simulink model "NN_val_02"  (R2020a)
settings: Solver=ode45  StartTime=0.0  StopTime=1000  RelTol=1e-3  EnableMultiTasking=on
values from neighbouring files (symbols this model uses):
  Ts = 0.05    [init_model.m]
libraries: neural x26

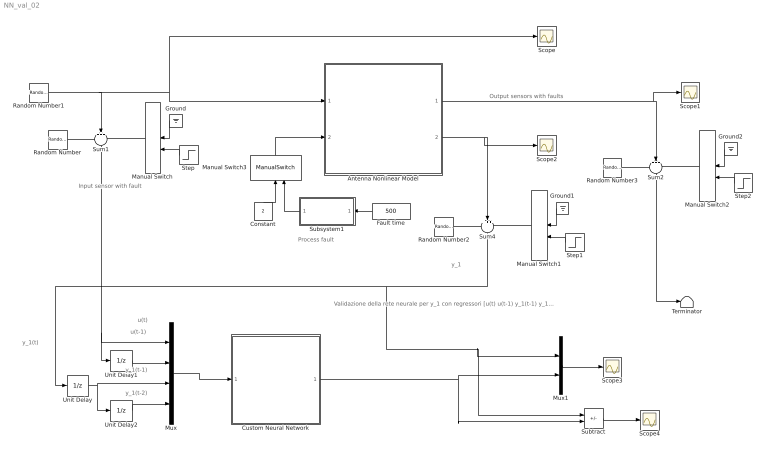
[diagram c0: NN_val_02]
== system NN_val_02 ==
  note: Validazione della rete neurale per y_1 con regressori [u(t) u(t-1) y_1(t-1) y_1(t-2)]
  note: y_1(t)
  note: y_1(t-1)
  note: y_1
  note: u(t)
  note: Output sensors with faults
  note: Process fault
  note: Input sensor with fault
  note: u(t-1)
  note: y_1(t-2)
  Antenna Nonlinear Model : Subsystem
  Constant : Constant  Value=2
  Custom Neural Network : Subsystem
      mask help: Custom Neural Network
  Fault time : Constant  Value=500
  Ground : Ground
  Ground1 : Ground
  Ground2 : Ground
  Manual Switch{,1..3} (4 alike) : ManualSwitch
  Mux : Mux
  Mux1 : Mux  Inputs=2
  Random Number : RandomNumber  Variance=0.0001  Seed=1  SampleTime=Ts
  Random Number1 : RandomNumber  Variance=0.1  SampleTime=10
  Random Number2 : RandomNumber  Variance=0.00001  Seed=2  SampleTime=Ts
  Random Number3 : RandomNumber  Variance=0.00001  Seed=3  SampleTime=Ts
  Scope{,1..4} (5 alike) : Scope
  Step : Step  Time=500  SampleTime=0
  Step1 : Step  Time=500  SampleTime=0
  Step2 : Step  Time=50  SampleTime=0
  Subsystem1 : Subsystem
  Subtract : Sum  Inputs=+-
  Sum1 : Sum  Inputs=+++  SaturateOnIntegerOverflow=on
  Sum2 : Sum  Inputs=+++  SaturateOnIntegerOverflow=on
  Sum4 : Sum  Inputs=+++  SaturateOnIntegerOverflow=on
  Terminator : Terminator
  Unit Delay : UnitDelay  SampleTime=Ts  HasFrameUpgradeWarning=on
  Unit Delay1 : UnitDelay  SampleTime=Ts  HasFrameUpgradeWarning=on
  Unit Delay2 : UnitDelay  SampleTime=Ts  HasFrameUpgradeWarning=on
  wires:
  Random Number1/1 -> Scope/1, Antenna Nonlinear Model/1(force), Sum1/2
  Random Number/1 -> Sum1/1
  Manual Switch/1 -> Sum1/3
  Sum1/1 -> Unit Delay1/1, Mux/1
  Ground/1 -> Manual Switch/1
  Step/1 -> Manual Switch/2
  Random Number2/1 -> Sum4/1
  Ground1/1 -> Manual Switch1/1
  Manual Switch1/1 -> Sum4/3
  Step1/1 -> Manual Switch1/2
  Antenna Nonlinear Model/2(velocity) -> Sum4/2, Scope2/1
  Random Number3/1 -> Sum2/1
  Ground2/1 -> Manual Switch2/1
  Manual Switch2/1 -> Sum2/3
  Step2/1 -> Manual Switch2/2
  Antenna Nonlinear Model/1(angle) -> Sum2/2, Scope1/1
  Sum2/1 -> Terminator/1
  Fault time/1 -> Subsystem1/1(Fault time)
  Subsystem1/1(Fault) -> Manual Switch3/2
  Manual Switch3/1 -> Antenna Nonlinear Model/2(drag)
  Constant/1 -> Manual Switch3/1
  Mux/1 -> Custom Neural Network/1(Input)
  Unit Delay1/1 -> Mux/2
  Unit Delay/1 -> Unit Delay2/1, Mux/3
  Unit Delay2/1 -> Mux/4
  Mux1/1 -> Scope3/1
  Custom Neural Network/1(Output) -> Subtract/2, Mux1/2
  Sum4/1 -> Mux1/1, Subtract/1, Unit Delay/1
  Subtract/1 -> Scope4/1

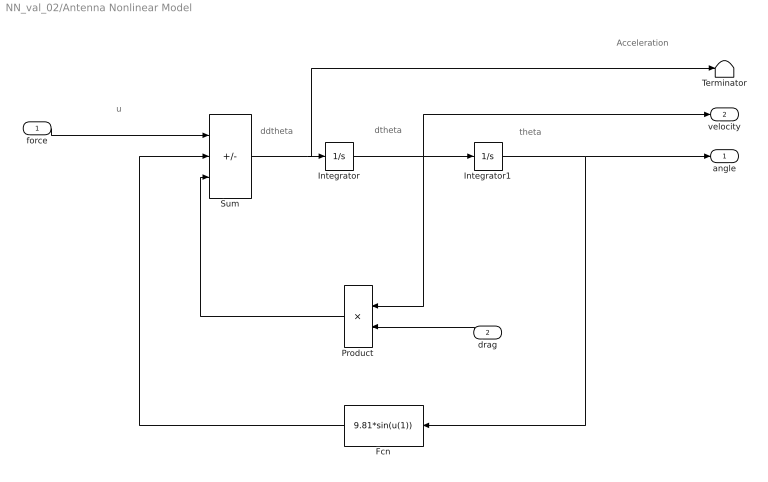
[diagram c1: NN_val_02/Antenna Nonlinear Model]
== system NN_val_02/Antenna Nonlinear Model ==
  note: Acceleration
  note: ddtheta
  note: dtheta
  note: theta
  note: u
  force : Inport
  drag : Inport  Port=2
  Fcn : Fcn  Expr=9.81*sin(u(1))
  Integrator : Integrator
  Integrator1 : Integrator  InitialCondition=(pi/180)*90
  Product : Product
  Sum : Sum  Inputs=+--  SaturateOnIntegerOverflow=on
  Terminator : Terminator
  angle : Outport
  velocity : Outport  Port=2
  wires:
  Sum/1 -> Terminator/1, Integrator/1
  Integrator/1 -> Product/1, Integrator1/1, velocity/1
  Integrator1/1 -> angle/1, Fcn/1
  Fcn/1 -> Sum/2
  Product/1 -> Sum/3
  force/1 -> Sum/1
  drag/1 -> Product/2

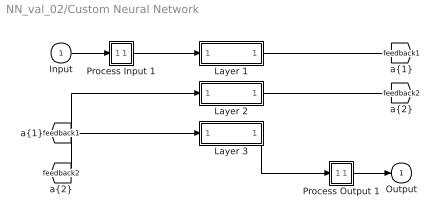
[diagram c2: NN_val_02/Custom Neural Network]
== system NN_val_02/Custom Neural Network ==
  Input : Inport  PortDimensions=4  SampleTime=0.05
  Layer 1 : Subsystem
  Layer 2 : Subsystem
  Layer 3 : Subsystem
  Process Input 1 : Subsystem
  Process Output 1 : Subsystem
  Output : Outport  InitialOutput=0
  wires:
  Input/1 -> Process Input 1/1(x)
  Process Output 1/1(y) -> Output/1
  Process Input 1/1(p) -> Layer 1/1("p{1}")
  Layer 1/1("a{1}") -> [feedback1]
  [feedback1] -> Layer 2/1("a{1} ")
  Layer 2/1("a{2}") -> [feedback2]
  [feedback2] -> Layer 3/1("a{2} ")
  Layer 3/1("a{3}") -> Process Output 1/1(a)

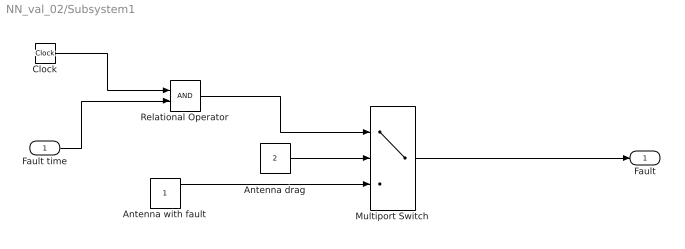
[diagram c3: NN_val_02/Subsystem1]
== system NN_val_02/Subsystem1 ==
  Fault time : Inport
  Antenna drag : Constant  Value=2
  Antenna with fault : Constant
  Clock : Clock
  Multiport Switch : MultiPortSwitch  DataPortOrder=Zero-based contiguous  Inputs=2  zeroidx=on
  Relational Operator : RelationalOperator  OutDataTypeStr=boolean  RndMeth=Simplest
  Fault : Outport
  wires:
  Clock/1 -> Relational Operator/1
  Fault time/1 -> Relational Operator/2
  Antenna drag/1 -> Multiport Switch/2
  Relational Operator/1 -> Multiport Switch/1
  Multiport Switch/1 -> Fault/1
  Antenna with fault/1 -> Multiport Switch/3

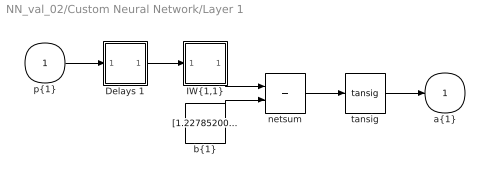
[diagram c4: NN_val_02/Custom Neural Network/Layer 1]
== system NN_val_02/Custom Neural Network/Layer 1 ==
  "p{1}" : Inport  PortDimensions=4  SampleTime=0.05
  Delays 1 : Subsystem
  "IW{1,1}" : Subsystem
  "b{1}" : Constant  Value=[1.227852000795871756366750560118816792964935302734375;-1.2068086972006153434477937480551190674304962158203125;-0.469116205279137721273485794881707988679409027099609375;0.537033543120907008727726861252449452877044677734375;0.68757712323574382562441087429760955274105072021484375;-2.165370420921475247411080999881960451602935791015625;-3.80990414820139111640173723571933805942535400390625]
  netsum : Sum  Inputs=2  InputSameDT=on  SaturateOnIntegerOverflow=on
  tansig : neural/Transfer Functions/tansig
  "a{1}" : Outport  InitialOutput=[0;0;0;0;0;0;0]
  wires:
  "p{1}"/1 -> Delays 1/1("p{1}")
  Delays 1/1("pd{1,1}") -> "IW{1,1}"/1("pd{1,1}")
  "IW{1,1}"/1("iz{1,1}") -> netsum/1
  "b{1}"/1 -> netsum/2
  netsum/1 -> tansig/1
  tansig/1 -> "a{1}"/1

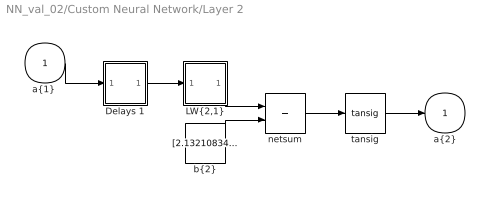
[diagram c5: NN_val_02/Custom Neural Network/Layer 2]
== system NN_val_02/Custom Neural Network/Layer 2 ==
  "a{1} " : Inport  PortDimensions=7  SampleTime=0.05
  Delays 1 : Subsystem
  "LW{2,1}" : Subsystem
  "b{2}" : Constant  Value=[2.132108348660313179578906783717684447765350341796875;2.220142305818061601030422025360167026519775390625;-1.5267770156364133260495918875676579773426055908203125;1.3641049967075142834715961726033128798007965087890625;0.80441149195895922385801668497151695191860198974609375;0.245980875629058015618966237525455653667449951171875;-0.5502430248009293478617109940387308597564697265625;0.187105156518366344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
  netsum : Sum  Inputs=2  InputSameDT=on  SaturateOnIntegerOverflow=on
  tansig : neural/Transfer Functions/tansig
  "a{2}" : Outport  InitialOutput=[0;0;0;0;0;0;0;0;0;0;0;0;0;0;0]
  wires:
  "a{1} "/1 -> Delays 1/1("p{2}")
  Delays 1/1("pd{2,1}") -> "LW{2,1}"/1("ad{2,1}")
  "LW{2,1}"/1("lz{2,1}") -> netsum/1
  "b{2}"/1 -> netsum/2
  netsum/1 -> tansig/1
  tansig/1 -> "a{2}"/1

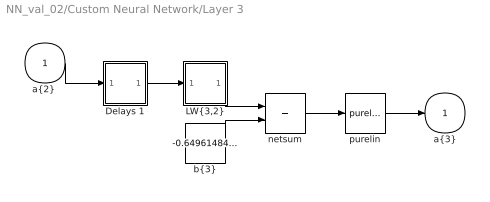
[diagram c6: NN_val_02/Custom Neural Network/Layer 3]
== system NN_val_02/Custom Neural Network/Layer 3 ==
  "a{2} " : Inport  PortDimensions=15  SampleTime=0.05
  Delays 1 : Subsystem
  "LW{3,2}" : Subsystem
  "b{3}" : Constant  Value=-0.64961484212074604993603088587406091392040252685546875
  netsum : Sum  Inputs=2  InputSameDT=on  SaturateOnIntegerOverflow=on
  purelin : neural/Transfer Functions/purelin
  "a{3}" : Outport  InitialOutput=0
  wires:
  "a{2} "/1 -> Delays 1/1("p{3}")
  Delays 1/1("pd{3,2}") -> "LW{3,2}"/1("ad{3,2}")
  "LW{3,2}"/1("lz{3,2}") -> netsum/1
  "b{3}"/1 -> netsum/2
  netsum/1 -> purelin/1
  purelin/1 -> "a{3}"/1

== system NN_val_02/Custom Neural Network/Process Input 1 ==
  x : Inport  PortDimensions=4  SampleTime=0.05
  p : Outport  PortDimensions=4  SampleTime=0.05
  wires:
  x/1 -> p/1

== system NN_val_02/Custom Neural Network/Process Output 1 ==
  a : Inport  PortDimensions=1  SampleTime=0.05
  y : Outport  PortDimensions=1  SampleTime=0.05
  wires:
  a/1 -> y/1

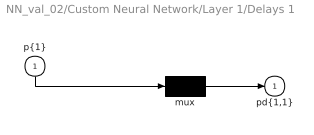
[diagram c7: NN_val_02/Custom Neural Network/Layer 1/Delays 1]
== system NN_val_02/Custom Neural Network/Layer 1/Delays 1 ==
  "p{1}" : Inport  PortDimensions=4  SampleTime=0.05
  mux : Mux  Inputs=1
  "pd{1,1}" : Outport
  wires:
  "p{1}"/1 -> mux/1
  mux/1 -> "pd{1,1}"/1

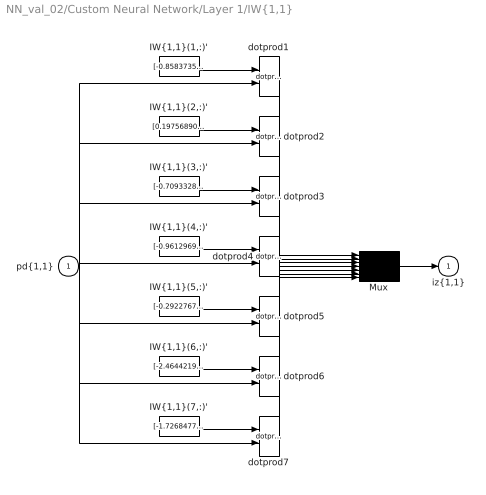
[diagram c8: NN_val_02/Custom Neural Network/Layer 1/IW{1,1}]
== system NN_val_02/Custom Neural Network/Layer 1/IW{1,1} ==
  "pd{1,1}" : Inport  PortDimensions=4  SampleTime=0.05
  "IW{1,1}(1,:)'" : Constant  Value=[-0.85837353691424123081077368624391965568065643310546875;-1.50167157946812235280731329112313687801361083984375;-1.2582699014576614882088279046001844108104705810546875;-0.81845080414747661823327007368789054453372955322265625]
  "IW{1,1}(2,:)'" : Constant  Value=[0.1975689051025306952613647126781870611011981964111328125;-1.1980691178201678948056496665230952203273773193359375;1.2091156479242730625855983817018568515777587890625;0.02637417164378029477145304326768382452428340911865234375]
  "IW{1,1}(3,:)'" : Constant  Value=[-0.7093328605358213412301893185940571129322052001953125;-2.107014242855214103400385283748619258403778076171875;-0.299913237321096204368586768396198749542236328125;-0.568643153566053438652261320385150611400604248046875]
  "IW{1,1}(4,:)'" : Constant  Value=[-0.96129696900881500543079027920612134039402008056640625;0.601804743455427892939724188181571662425994873046875;-0.7674148410687451349332377503742463886737823486328125;0.85896029266268880686396869350573979318141937255859375]
  "IW{1,1}(5,:)'" : Constant  Value=[-0.2922767950669269421126728047966025769710540771484375;0.2225160957405193096203532832078053615987300872802734375;0.8686197000875226503779913400649093091487884521484375;-0.279177521795706928831037885174737311899662017822265625]
  "IW{1,1}(6,:)'" : Constant  Value=[-2.464421946556701659147847749409265816211700439453125;-0.08884885706228863588851396571044460870325565338134765625;-0.27909020302141218650149312452413141727447509765625;0.422037319836571722664331218766164965927600860595703125]
  "IW{1,1}(7,:)'" : Constant  Value=[-1.7268477556460919419833999199909158051013946533203125;-0.1723568342494542215970199094954296015202999114990234375;-0.1833208379863790205011042644400731660425662994384765625;-0.6184209020560771374874775574426166713237762451171875]
  Mux : Mux  Inputs=7
  dotprod{1..7} (7 alike) : neural/Weight Functions/dotprod
  "iz{1,1}" : Outport
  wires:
  "IW{1,1}(1,:)'"/1 -> dotprod1/1
  "pd{1,1}"/1 -> dotprod1/2, dotprod2/2, dotprod3/2, dotprod4/2, dotprod5/2, dotprod6/2, dotprod7/2
  dotprod1/1 -> Mux/1
  "IW{1,1}(2,:)'"/1 -> dotprod2/1
  dotprod2/1 -> Mux/2
  "IW{1,1}(3,:)'"/1 -> dotprod3/1
  dotprod3/1 -> Mux/3
  "IW{1,1}(4,:)'"/1 -> dotprod4/1
  dotprod4/1 -> Mux/4
  "IW{1,1}(5,:)'"/1 -> dotprod5/1
  dotprod5/1 -> Mux/5
  "IW{1,1}(6,:)'"/1 -> dotprod6/1
  dotprod6/1 -> Mux/6
  "IW{1,1}(7,:)'"/1 -> dotprod7/1
  dotprod7/1 -> Mux/7
  Mux/1 -> "iz{1,1}"/1

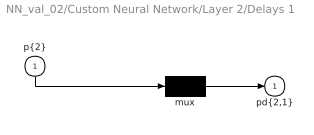
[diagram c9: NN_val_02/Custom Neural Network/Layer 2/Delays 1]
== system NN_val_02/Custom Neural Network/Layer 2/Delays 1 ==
  "p{2}" : Inport  PortDimensions=7  SampleTime=0.05
  mux : Mux  Inputs=1
  "pd{2,1}" : Outport
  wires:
  "p{2}"/1 -> mux/1
  mux/1 -> "pd{2,1}"/1

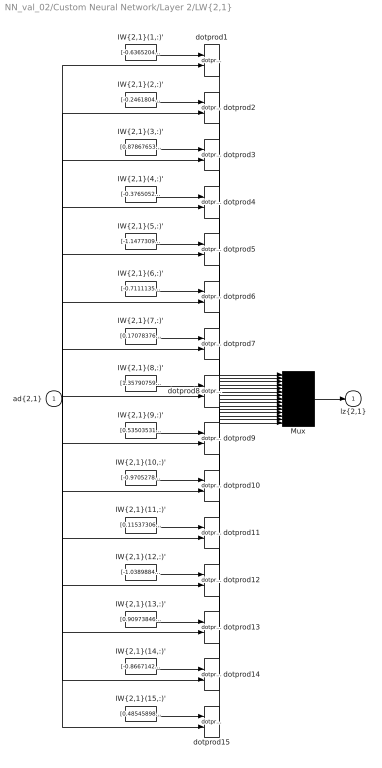
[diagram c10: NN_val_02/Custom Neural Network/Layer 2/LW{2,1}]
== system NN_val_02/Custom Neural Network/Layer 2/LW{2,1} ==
  "ad{2,1}" : Inport  PortDimensions=7  SampleTime=0.05
  "IW{2,1}(1,:)'" : Constant  Value=[-0.636520438499182272806820037658326327800750732421875;-0.92048078513578701631558942608535289764404296875;0.342189966413898705166474201178061775863170623779296875;-0.8071007452787510860758857234031893312931060791015625;0.308666465223191133215863146688207052648067474365234375;0.54860700642369975010836924411705695092678070068359375;-1.3452562754662638067060242974548600614070892333984375]
  "IW{2,1}(10,:)'" : Constant  Value=[-0.97052784094235955425489237313740886747837066650390625;-0.0501240179710435718174466046548332087695598602294921875;0.1727739851344505250807515039923600852489471435546875;0.94686942270448992697851053890190087258815765380859375;0.1812791919687547215200851269401027821004390716552734375;-0.5088052462981378365469709024182520806789398193359375;0.799020776260999099349646712653338909149169921875]
  "IW{2,1}(11,:)'" : Constant  Value=[0.11537306746287788461469148160176700912415981292724609375;-0.48294612937072012304184909226023592054843902587890625;-0.73224734868685470434712669884902425110340118408203125;1.1618122338537573146055592587799765169620513916015625;-1.001960528453451626518244665930978953838348388671875;0.3239302059936106648052600576193071901798248291015625;-0.98903819460521991135948383089271374046802520751953125]
  "IW{2,1}(12,:)'" : Constant  Value=[-1.0389884116270871050602409013663418591022491455078125;-0.026910750771055640118145646511038648895919322967529296875;-1.024908484176692002876052356441505253314971923828125;-0.272215779748138875238083755903062410652637481689453125;-1.021469491027882536826609793934039771556854248046875;0.7318960689388724905057870273594744503498077392578125;0.61280084425630843014687343384139239788055419921875]
  "IW{2,1}(13,:)'" : Constant  Value=[0.90973846629687005194142557229497469961643218994140625;0.2058345480427378471066646170584135688841342926025390625;0.06494946776615655170683538699449854902923107147216796875;-1.75712170340601137041858237353153526782989501953125;1.1330092097896964364878158448846079409122467041015625;-0.15539802412412384580164825820247642695903778076171875;0.1533727314316475354161184441181831061840057373046875]
  "IW{2,1}(14,:)'" : Constant  Value=[-0.86671422249502583223801366330008022487163543701171875;0.753579253233815027357422877685166895389556884765625;-0.8028756203769116250867909911903552711009979248046875;-0.62080212696188485921311439597047865390777587890625;-1.132320232661052639144827480777166783809661865234375;-0.44267131224761724350713620879105292260646820068359375;0.6116709115250633654881085021770559251308441162109375]
  "IW{2,1}(15,:)'" : Constant  Value=[0.485458982661166882355274765359354205429553985595703125;1.2593164923367492491479424643330276012420654296875;0.0963634945701961342923169695495744235813617706298828125;-0.475653158391175778785253669411758892238140106201171875;1.5626274683443879265354325980297289788722991943359375;0.71509144542904967689622708348906598985195159912109375;0.521217973749038332442751197959296405315399169921875]
  "IW{2,1}(2,:)'" : Constant  Value=[-0.2461804845936386432203590857170638628304004669189453125;-0.69718155527261005399708437835215590894222259521484375;-0.6322499918022044251841862205765210092067718505859375;-0.755024535371713767517576343379914760589599609375;-0.1794381511999492417874790817222674377262592315673828125;0.03282815460594638856672844440254266373813152313232421875;0.9100888276842920010523130258661694824695587158203125]
  "IW{2,1}(3,:)'" : Constant  Value=[0.87867653246198662575494608972803689539432525634765625;0.306263857973979813920095693902112543582916259765625;0.881753837966621656363486181362532079219818115234375;-0.923798161344731028066235012374818325042724609375;-0.008762454755530439676203258159148390404880046844482421875;0.08965807151409320441270978108150302432477474212646484375;1.2650919300093879105162386622396297752857208251953125]
  "IW{2,1}(4,:)'" : Constant  Value=[-0.376505262972612164684704794126446358859539031982421875;0.81507773475673117591355776312411762773990631103515625;-0.453377903062336107264940210370696149766445159912109375;-0.67783567601839334049174112806213088333606719970703125;0.493735040189397234033918948625796474516391754150390625;-0.81578104090500047629319624320487491786479949951171875;0.57923985108094522278321392150246538221836090087890625]
  "IW{2,1}(5,:)'" : Constant  Value=[-1.1477309344991117878720388034707866609096527099609375;-1.00285062391197943298948302981443703174591064453125;-0.524186838656582221318558367784135043621063232421875;-0.0477261627895378126584802203069557435810565948486328125;-0.630135077781108332573012376087717711925506591796875;-0.73916510557454417895684173345216549932956695556640625;-0.96077453781046517899966374898212961852550506591796875]
  "IW{2,1}(6,:)'" : Constant  Value=[-0.7111135038822664622415459234616719186305999755859375;1.032441357655538016757645891630090773105621337890625;1.2073698407589912307003032765351235866546630859375;0.412047115628940641141042533490690402686595916748046875;-1.2694711972943364397536925025633536279201507568359375;0.622872185754929308387772834976203739643096923828125;-0.1111094365057898325499508018765482120215892791748046875]
  "IW{2,1}(7,:)'" : Constant  Value=[0.170783763218426976049357790543581359088420867919921875;1.09084809888974376690384815447032451629638671875;0.6873217810395022553393573616631329059600830078125;1.182601075399613677063825889490544795989990234375;-0.3908165113089092645992650432162918150424957275390625;0.6700241338427510573438894425635226070880889892578125;-0.251911218512624712762004719479591585695743560791015625]
  "IW{2,1}(8,:)'" : Constant  Value=[1.3579075924959855825591148459352552890777587890625;-0.267325939258566569467490126044140197336673736572265625;0.41931735034773842674127308782772161066532135009765625;-0.6340934368757864536547685929690487682819366455078125;-0.83504114255150074797029446926899254322052001953125;-0.05247381933184940006054119976397487334907054901123046875;0.8536102070524778095972351366071961820125579833984375]
  "IW{2,1}(9,:)'" : Constant  Value=[0.53503531532991088770501164617598988115787506103515625;-0.2250225426213956769760926590606686659157276153564453125;0.4284118005158406017329753012745641171932220458984375;-1.0902982567582755191182286580442450940608978271484375;-0.275710404395244912389983937828219495713710784912109375;-0.93251153064707581474834796608774922788143157958984375;-1.258916495165529614297383886878378689289093017578125]
  Mux : Mux  Inputs=15
  dotprod{1..15} (15 alike) : neural/Weight Functions/dotprod
  "lz{2,1}" : Outport
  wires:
  "IW{2,1}(1,:)'"/1 -> dotprod1/1
  "ad{2,1}"/1 -> dotprod1/2, dotprod2/2, dotprod3/2, dotprod4/2, dotprod5/2, dotprod6/2, dotprod7/2, dotprod8/2, dotprod9/2, dotprod10/2, dotprod11/2, dotprod12/2, dotprod13/2, dotprod14/2, dotprod15/2
  dotprod1/1 -> Mux/1
  "IW{2,1}(2,:)'"/1 -> dotprod2/1
  dotprod2/1 -> Mux/2
  "IW{2,1}(3,:)'"/1 -> dotprod3/1
  dotprod3/1 -> Mux/3
  "IW{2,1}(4,:)'"/1 -> dotprod4/1
  dotprod4/1 -> Mux/4
  "IW{2,1}(5,:)'"/1 -> dotprod5/1
  dotprod5/1 -> Mux/5
  "IW{2,1}(6,:)'"/1 -> dotprod6/1
  dotprod6/1 -> Mux/6
  "IW{2,1}(7,:)'"/1 -> dotprod7/1
  dotprod7/1 -> Mux/7
  "IW{2,1}(8,:)'"/1 -> dotprod8/1
  dotprod8/1 -> Mux/8
  "IW{2,1}(9,:)'"/1 -> dotprod9/1
  dotprod9/1 -> Mux/9
  "IW{2,1}(10,:)'"/1 -> dotprod10/1
  dotprod10/1 -> Mux/10
  "IW{2,1}(11,:)'"/1 -> dotprod11/1
  dotprod11/1 -> Mux/11
  "IW{2,1}(12,:)'"/1 -> dotprod12/1
  dotprod12/1 -> Mux/12
  "IW{2,1}(13,:)'"/1 -> dotprod13/1
  dotprod13/1 -> Mux/13
  "IW{2,1}(14,:)'"/1 -> dotprod14/1
  dotprod14/1 -> Mux/14
  "IW{2,1}(15,:)'"/1 -> dotprod15/1
  dotprod15/1 -> Mux/15
  Mux/1 -> "lz{2,1}"/1

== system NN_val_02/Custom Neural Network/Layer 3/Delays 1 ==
  "p{3}" : Inport  PortDimensions=15  SampleTime=0.05
  mux : Mux  Inputs=1
  "pd{3,2}" : Outport
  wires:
  "p{3}"/1 -> mux/1
  mux/1 -> "pd{3,2}"/1

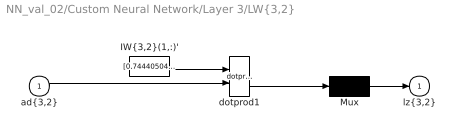
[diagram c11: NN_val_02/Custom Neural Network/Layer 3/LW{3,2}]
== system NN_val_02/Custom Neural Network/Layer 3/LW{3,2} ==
  "ad{3,2}" : Inport  PortDimensions=15  SampleTime=0.05
  "IW{3,2}(1,:)'" : Constant  Value=[0.74440504442132471307758123657549731433391571044921875;0.264656856737902124176997631366248242557048797607421875;-0.1874076515343474358399333823399501852691173553466796875;0.2398150923308920157150936347534297965466976165771484375;-0.77237807481697473566129019673098810017108917236328125;-0.76085104986466800536248911157599650323390960693359375;0.20024359110315032017624048421566840261220932006835937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
  Mux : Mux  Inputs=1
  dotprod1 : neural/Weight Functions/dotprod
  "lz{3,2}" : Outport
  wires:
  "IW{3,2}(1,:)'"/1 -> dotprod1/1
  "ad{3,2}"/1 -> dotprod1/2
  dotprod1/1 -> Mux/1
  Mux/1 -> "lz{3,2}"/1
